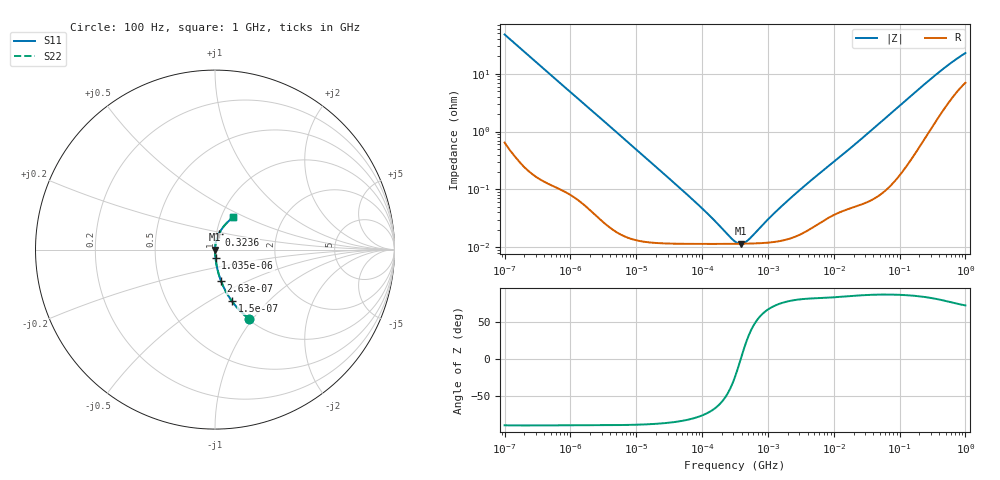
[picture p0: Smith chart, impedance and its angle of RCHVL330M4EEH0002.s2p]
! RCHVL330M4EEH0002  S-PARAMETER MODEL  (AEC-Q200 qualified)
! Model Generated by ELNA Corporation (http://www.ty-top.com)
! Version 1.0
! ELNA Control No. 231122
! Copyright (c) 2023 ELNA CO.,LTD. All Rights Reserved.
! Products Name : CONDUCTIVE POLYMER HYBRID ALUMINUM ELECTROLYTIC CAPACITORS
! Characteristics :
!  Capacitance  :  33uF  ,  Rated voltage  :  63V
!  Operating Temp. Range  :  -55 to +125 degC  ,  Endurance  :  8000hr at 125 degC
!  Dimension D  :  8mm  ,  Dimension L  :  10mm
! Frequency Range : 100Hz - 1GHz
! External Node Assignments :
!  1  o---| |---o  2
# MHz S RI R 50
!Freq[MHz].  S11 Real  S11 Imag  S21 Real  S21 Imag  S12 Real  S12 Imag  S22 Real  S22 Imag
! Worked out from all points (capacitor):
!   401 points, 100 Hz to 1 GHz, reference 50 ohm
!   read as one part in series: C = 33.4 uF near 108 Hz
!   lowest |Z| = 11.5 mohm at 386.8 kHz (marker M1)
!   series resonance near 386.7 kHz, so ESL is about 5.1 nH
!   S11 on the Smith chart (normalised r, x): 100 Hz: 1.01, -0.95; 150 Hz: 1.01, -0.64; 263 Hz: 1.00, -0.36; 1.035 kHz: 1.00, -0.09; 323.6 MHz: 1.03, +0.17; 1 GHz: 1.14, +0.43
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0.0001  0.1886 -0.3844  0.8114 0.3844  0.8114 0.3844  0.1886 -0.3844
0.00015  0.0948 -0.2876  0.9052 0.2876  0.9052 0.2876  0.0948 -0.2876
0.000263  0.0335 -0.1751  0.9665 0.1751  0.9665 0.1751  0.0335 -0.1751
0.000481  0.011 -0.0982  0.989 0.0982  0.989 0.0982  0.011 -0.0982
0.001035  0.00294 -0.0464  0.9971 0.0464  0.9971 0.0464  0.00294 -0.0464
0.001488  0.00164 -0.0325  0.9984 0.0325  0.9984 0.0325  0.00164 -0.0325
0.022131  0.000123 -0.00221  0.9999 0.00221  0.9999 0.00221  0.000123 -0.00221
0.098288  0.000115 -0.000466  0.9999 0.000466  0.9999 0.000466  0.000115 -0.000466
0.153109  0.000114 -0.00027  0.9999 0.00027  0.9999 0.00027  0.000114 -0.00027
0.269153  0.000115 -9.38e-05  0.9999 9.38e-05  0.9999 9.38e-05  0.000115 -9.38e-05
0.316228  0.000115 -5.13e-05  0.9999 5.13e-05  0.9999 5.13e-05  0.000115 -5.13e-05
0.386812  0.000115 9.4e-08  0.9999 -9.4e-08  0.9999 -9.4e-08  0.000115 9.4e-08
0.436516  0.000115 3.08e-05  0.9999 -3.08e-05  0.9999 -3.08e-05  0.000115 3.08e-05
0.512861  0.000116 7.25e-05  0.9999 -7.25e-05  0.9999 -7.25e-05  0.000116 7.25e-05
1.40443  0.000126 0.000423  0.9999 -0.000423  0.9999 -0.000423  0.000126 0.000423
4.704354  0.000219 0.00147  0.9998 -0.00147  0.9998 -0.00147  0.000219 0.00147
19.27525  0.000515 0.00551  0.9995 -0.00551  0.9995 -0.00551  0.000515 0.00551
69.9842  0.00149 0.0195  0.9985 -0.0195  0.9985 -0.0195  0.00149 0.0195
156.6751  0.00539 0.043  0.9946 -0.043  0.9946 -0.043  0.00539 0.043
323.5937  0.0198 0.0841  0.9802 -0.0841  0.9802 -0.0841  0.0198 0.0841
616.595  0.056 0.1383  0.944 -0.1383  0.944 -0.1383  0.056 0.1383
1000  0.102 0.1819  0.898 -0.1819  0.898 -0.1819  0.102 0.1819
